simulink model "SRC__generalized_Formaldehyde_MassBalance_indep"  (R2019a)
settings: Solver=VariableStepAuto  StartTime=0.0  StopTime=tend  RelTol=1e-3
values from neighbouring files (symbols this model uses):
  c_MeOH_0 = m_MeOH_sp_0/(m_MeOH_sp_0+m_air_sp_0)    [Mixer_script.m]
  comp_actuator_0 = [z0actuator,comp_w0]    [Compressor_script.m]
  comp_actuator_par = [comp_act_Ga;comp_act_tau;comp_act_zeta]    [Compressor_script.m]
  comp_deltaP = 2.1    [Compressor_script.m]
  comp_p1 = [a0,a1,a2,a3,b0,b1,b2,c0,c1,c2]    [Compressor_script.m]
  comp_p2 = [rho_a, kappa_a, cp_a, R_a, T_amb, d_c]    [Compressor_script.m]
  I_0_compressor = 0.39275    [Compressor_script.m]
  I_0_valve = valve_z0/valve_act_Ga    (= 0.7)    [Valve_script.m]
  Kc_comp = tau_compfotd/(K_compfotd*(tauc_comp+theta_compfotd))    [Compressor_script.m]
  Kc_mtot_MeOH = tau_mtot_MeOH/(K_mtot_MeOH*(tauc_mtot_MeOH+theta_mtot_MeOH))    (= 0.0903815050899)    [Basic_outer_PID_script.m]
  Kc_valve = tau_valvefotd/(K_valvefotd*(tauc_valve+theta_valvefotd))    [Valve_script.m]
  Kc_x_air = tau_x_air/(K_x_air*(tauc_x_air+theta_x_air))    (= -74361.4590706)    [Basic_outer_PID_script.m]
  KI_comp = Kc_comp/tauI_comp    [Compressor_script.m]
  KI_mtot_MeOH = Kc_mtot_MeOH/tauI_mtot_MeOH    [Basic_outer_PID_script.m]
  KI_SRC = Kc_SRC/tauI_SRC    [TuningSRC.m]
  KI_valve = Kc_valve/tauI_valve    [Valve_script.m]
  KI_x_air = Kc_x_air/tauI_x_air    [Basic_outer_PID_script.m]
  m_air_sp_0 = 23920    [Compressor_script.m]
  m_MeOH_sp_0 = 2940    [Valve_script.m]
  m_tot_sp_0 = m_air_sp_0+m_MeOH_sp_0    [main_VPC_formaldehyde.m]    (also in main_basic_formaldehyde.m; main_basicTPM_formaldehyde.m; main_SRC_formaldehyde.m)
  m_tot_sp_step1 = 0*m_tot_sp_0*0.15    [main_VPC_formaldehyde.m]    (also in main_basic_formaldehyde.m; main_basicTPM_formaldehyde.m; main_SRC_formaldehyde.m)
  m_tot_sp_step2 = 1*m_tot_sp_0*0.10    [main_VPC_formaldehyde.m]    (also in main_basic_formaldehyde.m; main_basicTPM_formaldehyde.m; main_SRC_formaldehyde.m)
  m_tot_sp_step3 = 0*(m_tot_sp_step2+m_tot_sp_step1)    [main_VPC_formaldehyde.m]    (also in main_basic_formaldehyde.m = -1*(m_tot_sp_step2+m_tot_sp_step1); main_basicTPM_formaldehyde.m = -1*(m_tot_sp_step2+m_tot_sp_step1); main_SRC_formaldehyde.m = -1*(m_tot_sp_step2+m_tot_sp_step1))
  m_tot_sp_step_t1 = 20    [main_VPC_formaldehyde.m]    (also in main_basic_formaldehyde.m; main_basicTPM_formaldehyde.m; main_SRC_formaldehyde.m)
  m_tot_sp_step_t2 = 30    [main_VPC_formaldehyde.m]    (also in main_basic_formaldehyde.m; main_basicTPM_formaldehyde.m; main_SRC_formaldehyde.m)
  m_tot_sp_step_t3 = 60    [main_VPC_formaldehyde.m]    (also in main_basic_formaldehyde.m = 70; main_basicTPM_formaldehyde.m = 70; main_SRC_formaldehyde.m = 70)
  max_air_PI = mair_max-m_air_sp_0    [Basic_outer_PID_script.m]
  max_MeOH_PI = m_MeOH_max-m_MeOH_sp_0    [Basic_outer_PID_script.m]
  min_air_PI = mair_min-m_air_sp_0    [Basic_outer_PID_script.m]
  min_MeOH_PI = m_MeOH_min-m_MeOH_sp_0    [Basic_outer_PID_script.m]
  N_cmax = 10048    [Compressor_script.m]
  N_cmin = 7500    [Compressor_script.m]
  p_mix = [MW_MeOH;MW_air;rho_MeOH;rho_a;V_mixer]    [Mixer_script.m]
  PI_comp_max = 0.2    [Compressor_script.m]
  PI_comp_min = -I_0_compressor    (= -0.39275)    [Compressor_script.m]
  type_of_bias = 1    [main_SRC_formaldehyde.m]
  valve_actuator_0 = [valve_z0 valve_w0]    [Valve_script.m]
  valve_actuator_par = [valve_act_Ga;valve_act_tau;valve_act_zeta]    [Valve_script.m]
  valve_Cv = m_MeOH_max/sqrt(valve_delta_p)    [Valve_script.m]
  valve_delta_p = 0.5    [Valve_script.m]
  valve_type = 3    [Valve_script.m]
  x_MeOH_sp_step1 = 1*-0.005    (= -0.005)    [main_VPC_formaldehyde.m]    (also in main_basic_formaldehyde.m; main_basicTPM_formaldehyde.m; main_SRC_formaldehyde.m)
  x_MeOH_sp_step2 = 0*-0.005    (= 0)    [main_VPC_formaldehyde.m]    (also in main_basic_formaldehyde.m; main_basicTPM_formaldehyde.m; main_SRC_formaldehyde.m)
  x_MeOH_sp_step3 = 0*+0.01    (= 0)    [main_VPC_formaldehyde.m]    (also in main_basic_formaldehyde.m; main_basicTPM_formaldehyde.m; main_SRC_formaldehyde.m)
  x_MeOH_sp_step_t1 = 10    [main_VPC_formaldehyde.m]    (also in main_basic_formaldehyde.m; main_basicTPM_formaldehyde.m; main_SRC_formaldehyde.m)
  x_MeOH_sp_step_t2 = 40    [main_VPC_formaldehyde.m]    (also in main_basic_formaldehyde.m; main_basicTPM_formaldehyde.m; main_SRC_formaldehyde.m)
  x_MeOH_sp_step_t3 = 60    [main_VPC_formaldehyde.m]    (also in main_basic_formaldehyde.m = 70; main_basicTPM_formaldehyde.m = 70; main_SRC_formaldehyde.m = 70)
  x_MeOHsp_0 = 0.1    [main_VPC_formaldehyde.m]    (also in main_basic_formaldehyde.m; main_basicTPM_formaldehyde.m; main_SRC_formaldehyde.m)
undefined symbols (not defined in the file or in its folder): actuator, Bias_calc, Bias_par, compressor, Kc_air, Kc_MeOH, KI_MeOH, m_MeOH_bias_constant, mixerMeOH_O2_dynamic, mixerMeOH_O2_ss, SRC_par, valve
libraries: simulink x5

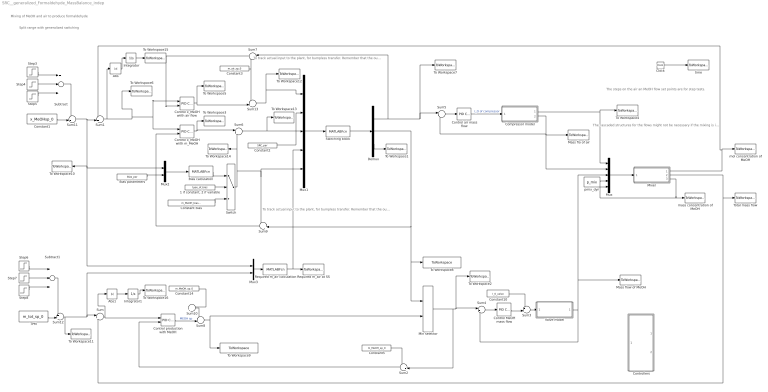
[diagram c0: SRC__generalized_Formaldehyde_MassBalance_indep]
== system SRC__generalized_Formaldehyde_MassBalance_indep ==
  note: Mixing of MeOH and air to produce formaldehyde
  note: The cascaded structures for the flows might not be necessary if the mixing is instantaneous. I just added them to have a general structure. I also added a small residence time in the tank.
  note: The steps on the air an MeOH flow set points are for step tests.
  note: Split range with generalized switching
  note: To track actual input to the plant, for bumpless transfer. Remember that the output of the PI is in deviaton, substract bias.
  note: To track actual input to the plant, for bumpless transfer. Remember that the output of the PI is in deviaton, substract bias.
  "1 if constant, 2 if variable" : Constant  Value=type_of_bias
  Abs : Abs
  Abs1 : Abs
  Bias calculation : MATLABFcn  MATLABFcn=Bias_calc(u)
  Bias parameters : Constant  Value=Bias_par
  Clock : Clock
  Compressor model : Subsystem
  Constant bias : Constant  Value=m_MeOH_bias_constant
  Constant1 : Constant  Value=x_MeOHsp_0
  Constant10 : Constant  Value=I_0_valve
  Constant14 : Constant  Value=m_MeOH_sp_0
  Constant2 : Constant  Value=SRC_par
  Constant3 : Constant  Value=m_air_sp_0
  Constant5 : Constant  Value=m_MeOH_sp_0
  Control MeOH mass flow : simulink/Continuous/PID Controller  Controller=PI  Form=Parallel  TimeDomain=Continuous-time  SampleTime=-1  IntegratorMethod=Forward Euler  FilterMethod=Forward Euler  ControllerParametersSource=internal  P=Kc_valve  I=KI_valve  D=0  UseFilter=on  N=100  TunerSelectOption=Transfer Function Based (PID Tuner App)  InitialConditionSource=internal  InitialConditionForIntegrator=0  InitialConditionForFilter=0  DifferentiatorICPrevScaledInput=0  ExternalReset=none  TrackingMode=off  Kt=1  LimitOutput=on  UpperSaturationLimit=1-I_0_valve  LowerSaturationLimit=-I_0_valve  LinearizeAsGain=on  AntiWindupMode=back-calculation  Kb=1  POutMin=[]  POutMax=[]  IOutMin=[]  IOutMax=[]  DOutMin=[]  DOutMax=[]  NOutMin=[]  NOutMax=[]  SumOutMin=[]  SumOutMax=[]  SaturationOutMin=[]  SaturationOutMax=[]  PParamMin=[]  PParamMax=[]  IParamMin=[]  IParamMax=[]  DParamMin=[]  DParamMax=[]  NParamMin=[]  NParamMax=[]  KbParamMin=[]  KbParamMax=[]  KtParamMin=[]  KtParamMax=[]  KbOutMin=[]  KbOutMax=[]  KtOutMin=[]  KtOutMax=[]  IntegratorOutMin=[]  IntegratorOutMax=[]  FilterOutMin=[]  FilterOutMax=[]  SumI1OutMin=[]  SumI1OutMax=[]  SumI2OutMin=[]  SumI2OutMax=[]  SumI3OutMin=[]  SumI3OutMax=[]  SumI4OutMin=[]  SumI4OutMax=[]  SumDOutMin=[]  SumDOutMax=[]  DifferentiatorOutMin=[]  DifferentiatorOutMax=[]  FilterDiffOutCoefMin=[]  FilterDiffOutCoefMax=[]  ReciprocalOutMin=[]  ReciprocalOutMax=[]  SumDenOutMin=[]  SumDenOutMax=[]  SumNumOutMin=[]  SumNumOutMax=[]  DivideOutMin=[]  DivideOutMax=[]  IntegratorContinuousStateAttributes=''  IntegratorStateMustResolveToSignalObject=off  IntegratorRTWStateStorageClass=Auto  FilterContinuousStateAttributes=''  FilterStateMustResolveToSignalObject=off  FilterRTWStateStorageClass=Auto  ParallelPVariant=InternalParameters  IdealPVariant=Disabled  IVariant=InternalParameters  DVariant=Disabled  IntegratorVariant=Continuous  SatVariant=Enabled  AWVariant=BackCalculation  PCopyVariant=Disabled  TRVariant=Disabled  FdbkBlocksVariant=Forward  IdealPFdbkVariant=Disabled  SatFdbkVariant=Disabled  DerivativeFilterVariant=Disabled  NVariant=Disabled  NCopyVariant=Disabled_SignalSpec  FilterICVariant=Disabled  IntegratorICVariant=InternalICs  ExternalResetVariant=Disabled  TRSumVariant=Passthrough  SumFdbkVariant=Disabled  SumVariant=Sum_PI
  Control air mass flow : simulink/Continuous/PID Controller  Controller=PI  Form=Parallel  TimeDomain=Continuous-time  SampleTime=-1  IntegratorMethod=Forward Euler  FilterMethod=Forward Euler  ControllerParametersSource=internal  P=Kc_comp  I=KI_comp  D=0  UseFilter=on  N=100  TunerSelectOption=Transfer Function Based (PID Tuner App)  InitialConditionSource=internal  InitialConditionForIntegrator=0  InitialConditionForFilter=0  DifferentiatorICPrevScaledInput=0  ExternalReset=none  TrackingMode=off  Kt=1  LimitOutput=on  UpperSaturationLimit=PI_comp_max  LowerSaturationLimit=PI_comp_min  LinearizeAsGain=on  AntiWindupMode=back-calculation  Kb=1  POutMin=[]  POutMax=[]  IOutMin=[]  IOutMax=[]  DOutMin=[]  DOutMax=[]  NOutMin=[]  NOutMax=[]  SumOutMin=[]  SumOutMax=[]  SaturationOutMin=[]  SaturationOutMax=[]  PParamMin=[]  PParamMax=[]  IParamMin=[]  IParamMax=[]  DParamMin=[]  DParamMax=[]  NParamMin=[]  NParamMax=[]  KbParamMin=[]  KbParamMax=[]  KtParamMin=[]  KtParamMax=[]  KbOutMin=[]  KbOutMax=[]  KtOutMin=[]  KtOutMax=[]  IntegratorOutMin=[]  IntegratorOutMax=[]  FilterOutMin=[]  FilterOutMax=[]  SumI1OutMin=[]  SumI1OutMax=[]  SumI2OutMin=[]  SumI2OutMax=[]  SumI3OutMin=[]  SumI3OutMax=[]  SumI4OutMin=[]  SumI4OutMax=[]  SumDOutMin=[]  SumDOutMax=[]  DifferentiatorOutMin=[]  DifferentiatorOutMax=[]  FilterDiffOutCoefMin=[]  FilterDiffOutCoefMax=[]  ReciprocalOutMin=[]  ReciprocalOutMax=[]  SumDenOutMin=[]  SumDenOutMax=[]  SumNumOutMin=[]  SumNumOutMax=[]  DivideOutMin=[]  DivideOutMax=[]  IntegratorContinuousStateAttributes=''  IntegratorStateMustResolveToSignalObject=off  IntegratorRTWStateStorageClass=Auto  FilterContinuousStateAttributes=''  FilterStateMustResolveToSignalObject=off  FilterRTWStateStorageClass=Auto  ParallelPVariant=InternalParameters  IdealPVariant=Disabled  IVariant=InternalParameters  DVariant=Disabled  IntegratorVariant=Continuous  SatVariant=Enabled  AWVariant=BackCalculation  PCopyVariant=Disabled  TRVariant=Disabled  FdbkBlocksVariant=Forward  IdealPFdbkVariant=Disabled  SatFdbkVariant=Disabled  DerivativeFilterVariant=Disabled  NVariant=Disabled  NCopyVariant=Disabled_SignalSpec  FilterICVariant=Disabled  IntegratorICVariant=InternalICs  ExternalResetVariant=Disabled  TRSumVariant=Passthrough  SumFdbkVariant=Disabled  SumVariant=Sum_PI
  Control production with MeOH : simulink/Continuous/PID Controller  Controller=PI  Form=Parallel  TimeDomain=Continuous-time  SampleTime=-1  IntegratorMethod=Forward Euler  FilterMethod=Forward Euler  ControllerParametersSource=internal  P=Kc_mtot_MeOH  I=KI_mtot_MeOH  D=0  UseFilter=on  N=100  TunerSelectOption=Transfer Function Based (PID Tuner App)  InitialConditionSource=internal  InitialConditionForIntegrator=0  InitialConditionForFilter=0  DifferentiatorICPrevScaledInput=0  ExternalReset=none  TrackingMode=on  Kt=1  LimitOutput=on  UpperSaturationLimit=max_MeOH_PI  LowerSaturationLimit=min_MeOH_PI  LinearizeAsGain=on  AntiWindupMode=back-calculation  Kb=1  POutMin=[]  POutMax=[]  IOutMin=[]  IOutMax=[]  DOutMin=[]  DOutMax=[]  NOutMin=[]  NOutMax=[]  SumOutMin=[]  SumOutMax=[]  SaturationOutMin=[]  SaturationOutMax=[]  PParamMin=[]  PParamMax=[]  IParamMin=[]  IParamMax=[]  DParamMin=[]  DParamMax=[]  NParamMin=[]  NParamMax=[]  KbParamMin=[]  KbParamMax=[]  KtParamMin=[]  KtParamMax=[]  KbOutMin=[]  KbOutMax=[]  KtOutMin=[]  KtOutMax=[]  IntegratorOutMin=[]  IntegratorOutMax=[]  FilterOutMin=[]  FilterOutMax=[]  SumI1OutMin=[]  SumI1OutMax=[]  SumI2OutMin=[]  SumI2OutMax=[]  SumI3OutMin=[]  SumI3OutMax=[]  SumI4OutMin=[]  SumI4OutMax=[]  SumDOutMin=[]  SumDOutMax=[]  DifferentiatorOutMin=[]  DifferentiatorOutMax=[]  FilterDiffOutCoefMin=[]  FilterDiffOutCoefMax=[]  ReciprocalOutMin=[]  ReciprocalOutMax=[]  SumDenOutMin=[]  SumDenOutMax=[]  SumNumOutMin=[]  SumNumOutMax=[]  DivideOutMin=[]  DivideOutMax=[]  IntegratorContinuousStateAttributes=''  IntegratorStateMustResolveToSignalObject=off  IntegratorRTWStateStorageClass=Auto  FilterContinuousStateAttributes=''  FilterStateMustResolveToSignalObject=off  FilterRTWStateStorageClass=Auto  ParallelPVariant=InternalParameters  IdealPVariant=Disabled  IVariant=InternalParameters  DVariant=Disabled  IntegratorVariant=Continuous  SatVariant=Enabled  AWVariant=BackCalculation  PCopyVariant=Disabled  TRVariant=Enabled  FdbkBlocksVariant=Forward  IdealPFdbkVariant=Disabled  SatFdbkVariant=Disabled  DerivativeFilterVariant=Disabled  NVariant=Disabled  NCopyVariant=Disabled_SignalSpec  FilterICVariant=Disabled  IntegratorICVariant=InternalICs  ExternalResetVariant=Disabled  TRSumVariant=TrackingMode  SumFdbkVariant=Disabled  SumVariant=Sum_PI
  Control x_MeOH wiith air flow : simulink/Continuous/PID Controller  Controller=PI  Form=Parallel  TimeDomain=Continuous-time  SampleTime=-1  IntegratorMethod=Forward Euler  FilterMethod=Forward Euler  ControllerParametersSource=internal  P=Kc_x_air  I=KI_x_air  D=0  UseFilter=on  N=100  TunerSelectOption=Transfer Function Based (PID Tuner App)  InitialConditionSource=internal  InitialConditionForIntegrator=0  InitialConditionForFilter=0  DifferentiatorICPrevScaledInput=0  ExternalReset=none  TrackingMode=on  Kt=1  LimitOutput=on  UpperSaturationLimit=max_air_PI  LowerSaturationLimit=min_air_PI  LinearizeAsGain=on  AntiWindupMode=back-calculation  Kb=1  POutMin=[]  POutMax=[]  IOutMin=[]  IOutMax=[]  DOutMin=[]  DOutMax=[]  NOutMin=[]  NOutMax=[]  SumOutMin=[]  SumOutMax=[]  SaturationOutMin=[]  SaturationOutMax=[]  PParamMin=[]  PParamMax=[]  IParamMin=[]  IParamMax=[]  DParamMin=[]  DParamMax=[]  NParamMin=[]  NParamMax=[]  KbParamMin=[]  KbParamMax=[]  KtParamMin=[]  KtParamMax=[]  KbOutMin=[]  KbOutMax=[]  KtOutMin=[]  KtOutMax=[]  IntegratorOutMin=[]  IntegratorOutMax=[]  FilterOutMin=[]  FilterOutMax=[]  SumI1OutMin=[]  SumI1OutMax=[]  SumI2OutMin=[]  SumI2OutMax=[]  SumI3OutMin=[]  SumI3OutMax=[]  SumI4OutMin=[]  SumI4OutMax=[]  SumDOutMin=[]  SumDOutMax=[]  DifferentiatorOutMin=[]  DifferentiatorOutMax=[]  FilterDiffOutCoefMin=[]  FilterDiffOutCoefMax=[]  ReciprocalOutMin=[]  ReciprocalOutMax=[]  SumDenOutMin=[]  SumDenOutMax=[]  SumNumOutMin=[]  SumNumOutMax=[]  DivideOutMin=[]  DivideOutMax=[]  IntegratorContinuousStateAttributes=''  IntegratorStateMustResolveToSignalObject=off  IntegratorRTWStateStorageClass=Auto  FilterContinuousStateAttributes=''  FilterStateMustResolveToSignalObject=off  FilterRTWStateStorageClass=Auto  ParallelPVariant=InternalParameters  IdealPVariant=Disabled  IVariant=InternalParameters  DVariant=Disabled  IntegratorVariant=Continuous  SatVariant=Enabled  AWVariant=BackCalculation  PCopyVariant=Disabled  TRVariant=Enabled  FdbkBlocksVariant=Forward  IdealPFdbkVariant=Disabled  SatFdbkVariant=Disabled  DerivativeFilterVariant=Disabled  NVariant=Disabled  NCopyVariant=Disabled_SignalSpec  FilterICVariant=Disabled  IntegratorICVariant=InternalICs  ExternalResetVariant=Disabled  TRSumVariant=TrackingMode  SumFdbkVariant=Disabled  SumVariant=Sum_PI
  Control x_MeOH wiith m_MeOH : simulink/Continuous/PID Controller  Controller=PI  Form=Parallel  TimeDomain=Continuous-time  SampleTime=-1  IntegratorMethod=Forward Euler  FilterMethod=Forward Euler  ControllerParametersSource=internal  P=Kc_MeOH  I=KI_MeOH  D=0  UseFilter=on  N=100  TunerSelectOption=Transfer Function Based (PID Tuner App)  InitialConditionSource=internal  InitialConditionForIntegrator=0  InitialConditionForFilter=0  DifferentiatorICPrevScaledInput=0  ExternalReset=none  TrackingMode=on  Kt=1  LimitOutput=on  UpperSaturationLimit=inf  LowerSaturationLimit=-inf  LinearizeAsGain=on  AntiWindupMode=back-calculation  Kb=1  POutMin=[]  POutMax=[]  IOutMin=[]  IOutMax=[]  DOutMin=[]  DOutMax=[]  NOutMin=[]  NOutMax=[]  SumOutMin=[]  SumOutMax=[]  SaturationOutMin=[]  SaturationOutMax=[]  PParamMin=[]  PParamMax=[]  IParamMin=[]  IParamMax=[]  DParamMin=[]  DParamMax=[]  NParamMin=[]  NParamMax=[]  KbParamMin=[]  KbParamMax=[]  KtParamMin=[]  KtParamMax=[]  KbOutMin=[]  KbOutMax=[]  KtOutMin=[]  KtOutMax=[]  IntegratorOutMin=[]  IntegratorOutMax=[]  FilterOutMin=[]  FilterOutMax=[]  SumI1OutMin=[]  SumI1OutMax=[]  SumI2OutMin=[]  SumI2OutMax=[]  SumI3OutMin=[]  SumI3OutMax=[]  SumI4OutMin=[]  SumI4OutMax=[]  SumDOutMin=[]  SumDOutMax=[]  DifferentiatorOutMin=[]  DifferentiatorOutMax=[]  FilterDiffOutCoefMin=[]  FilterDiffOutCoefMax=[]  ReciprocalOutMin=[]  ReciprocalOutMax=[]  SumDenOutMin=[]  SumDenOutMax=[]  SumNumOutMin=[]  SumNumOutMax=[]  DivideOutMin=[]  DivideOutMax=[]  IntegratorContinuousStateAttributes=''  IntegratorStateMustResolveToSignalObject=off  IntegratorRTWStateStorageClass=Auto  FilterContinuousStateAttributes=''  FilterStateMustResolveToSignalObject=off  FilterRTWStateStorageClass=Auto  ParallelPVariant=InternalParameters  IdealPVariant=Disabled  IVariant=InternalParameters  DVariant=Disabled  IntegratorVariant=Continuous  SatVariant=Enabled  AWVariant=BackCalculation  PCopyVariant=Disabled  TRVariant=Enabled  FdbkBlocksVariant=Forward  IdealPFdbkVariant=Disabled  SatFdbkVariant=Disabled  DerivativeFilterVariant=Disabled  NVariant=Disabled  NCopyVariant=Disabled_SignalSpec  FilterICVariant=Disabled  IntegratorICVariant=InternalICs  ExternalResetVariant=Disabled  TRSumVariant=TrackingMode  SumFdbkVariant=Disabled  SumVariant=Sum_PI
  Controllers : Subsystem
  Demux : Demux  Outputs=3
  Integrator : Integrator
  Integrator1 : Integrator
  Mass flo of air : ToWorkspace  VariableName=m_air  SampleTime=-1
  Mass flow of MeOH : ToWorkspace  VariableName=m_MeOH  SampleTime=-1
  Min selector : MinMax  Inputs=2
  Mixer : Subsystem
  Mux : Mux  Inputs=5
  Mux1 : Mux  Inputs=5
  Mux2 : Mux  Inputs=2
  Mux3 : Mux  Inputs=2
  Required m_air at SS : ToWorkspace  VariableName=m_air_req  SampleTime=-1
  Required m_air calculation : MATLABFcn  MATLABFcn=Required_mair  OutputDimensions=1
  Step3 : Step  Time=x_MeOH_sp_step_t1  After=x_MeOH_sp_step1  SampleTime=0
  Step4 : Step  Time=x_MeOH_sp_step_t2  After=x_MeOH_sp_step2  SampleTime=0
  Step5 : Step  Time=x_MeOH_sp_step_t3  After=x_MeOH_sp_step3  SampleTime=0
  Step6 : Step  Time=m_tot_sp_step_t1  After=m_tot_sp_step1  SampleTime=0
  Step7 : Step  Time=m_tot_sp_step_t2  After=m_tot_sp_step2  SampleTime=0
  Step8 : Step  Time=m_tot_sp_step_t3  After=m_tot_sp_step3  SampleTime=0
  Subtract : Sum  Inputs=+++
  Subtract1 : Sum  Inputs=+++
  Sum{,4..5,7} (4 alike) : Sum  Inputs=|+-
  Sum1 : Sum  Inputs=-+|
  Sum{3,8,10..13} (6 alike) : Sum  Inputs=++|
  Sum2 : Sum  Inputs=-+|
  Sum6 : Sum  Inputs=|++
  Sum9 : Sum  Inputs=-+|
  Switch : Switch  Criteria=u2 > Threshold  Threshold=1
  Switching block : MATLABFcn  MATLABFcn=SR_switch2_MassBalance  OutputDimensions=3
  TPM : Constant  Value=m_tot_sp_0
  To Workspace1 : ToWorkspace  VariableName=activeMV  SampleTime=-1
  To Workspace10 : ToWorkspace  VariableName=x_MeOHsp  SampleTime=-1
  To Workspace11 : ToWorkspace  VariableName=m_tot_sp  SampleTime=-1
  To Workspace12 : ToWorkspace  VariableName=u_air  SampleTime=-1
  To Workspace13 : ToWorkspace  VariableName=u_MeOH  SampleTime=-1
  To Workspace14 : ToWorkspace  VariableName=bias_MeOH  SampleTime=-1
  To Workspace15 : ToWorkspace  VariableName=IAE_xMeOH  SampleTime=-1
  To Workspace16 : ToWorkspace  VariableName=IAE_mtot  SampleTime=-1
  To Workspace2 : ToWorkspace  VariableName=m_MEOH_sp  SampleTime=-1
  To Workspace3 : ToWorkspace  VariableName=v_MeOH  SampleTime=-1
  To Workspace4 : ToWorkspace  VariableName=Q_air  SampleTime=-1
  To Workspace5 : ToWorkspace  VariableName=v_air  SampleTime=-1
  To Workspace6 : ToWorkspace  VariableName=x_MeOH_error  SampleTime=-1
  To Workspace7 : ToWorkspace  VariableName=m_air_sp  SampleTime=-1
  To Workspace8 : ToWorkspace  VariableName=m_MEOH_sp_SR  SampleTime=-1
  To Workspace9 : ToWorkspace  VariableName=m_MeOH_sp_m_tot  SampleTime=-1
  Total mass flow : ToWorkspace  VariableName=m_tot  SampleTime=-1
  Valve model : Subsystem
  mass concentration of MeOH : ToWorkspace  VariableName=c_MeOH  SampleTime=-1
  mol concentration of MeOH : ToWorkspace  VariableName=x_MeOH  SampleTime=-1
  pmix_dyn : Constant  Value=p_mix
  time : ToWorkspace  VariableName=t  SampleTime=-1
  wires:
  Valve model/1(m_MeOH) -> Mass flow of MeOH/1, Mux/3, Sum4/2
  Clock/1 -> time/1
  Compressor model/2(m_air) -> Sum5/2, Mux/2, Mass flo of air/1
  Compressor model/1(Q_air) -> Mux/1, To Workspace4/1
  Control MeOH mass flow/1 -> Sum3/2
  Constant10/1 -> Sum3/1
  Sum4/1 -> Control MeOH mass flow/1
  Mixer/2(m_tot) -> Total mass flow/1, Sum/2
  Mixer/1(x_MeOH) -> Sum1/1, mol concentration of MeOH/1
  pmix_dyn/1 -> Mux/4
  Sum10/1 -> Sum8/1
  Constant1/1 -> Sum11/2
  Sum11/1 -> Mux3/1, Mux2/1, To Workspace10/1, Sum1/2
  Step3/1 -> Subtract/1
  Step4/1 -> Subtract/2
  Step5/1 -> Subtract/3
  TPM/1 -> Sum12/2
  Sum12/1 -> To Workspace11/1, Mux3/2, Sum/1
  Step6/1 -> Subtract1/1
  Step7/1 -> Subtract1/2
  Step8/1 -> Subtract1/3
  Subtract1/1 -> Sum12/1
  Sum1/1 -> Abs/1, Control x_MeOH wiith m_MeOH/1, Control x_MeOH wiith air flow/1, To Workspace6/1
  Control air mass flow/1 -> Compressor model/1(I_blower)  "I_O of compressor"
  Sum5/1 -> Control air mass flow/1
  Mux/1 -> Mixer/1(Mix_par)
  Mixer/3(c_MeOH) -> Mux/5, mass concentration of MeOH/1
  Sum3/1 -> Valve model/1(I_valve)
  Mux1/1 -> Switching block/1
  Control x_MeOH wiith air flow/1 -> Sum13/2, To Workspace5/1
  Control x_MeOH wiith m_MeOH/1 -> To Workspace3/1, Sum6/1
  Switching block/1 -> Demux/1
  Demux/3 -> To Workspace1/1
  Demux/2 -> Sum9/2, Min selector/1, To Workspace8/1
  Sum/1 -> Abs1/1, Control production with MeOH/1
  Sum8/1 -> To Workspace9/1, Min selector/2
  Min selector/1 -> Sum2/2, To Workspace2/1, Sum4/1
  Sum13/1 -> To Workspace12/1, Mux1/1
  Constant3/1 -> Sum13/1, Sum7/2
  Sum6/1 -> To Workspace13/1, Mux1/2
  Constant2/1 -> Mux1/3
  Constant14/1 -> Sum10/1
  Constant bias/1 -> Switch/3
  Switch/1 -> Mux1/5, Sum9/1, To Workspace14/1, Sum6/2
  "1 if constant, 2 if variable"/1 -> Switch/2
  Bias calculation/1 -> Switch/1
  Mux2/1 -> Bias calculation/1
  Bias parameters/1 -> Mux2/2
  Demux/1 -> Sum7/1, To Workspace7/1, Sum5/1
  Control production with MeOH/1 -> Sum8/2  "MEOH sp"
  Subtract/1 -> Sum11/1
  Required m_air calculation/1 -> Required m_air at SS/1, Mux1/4
  Mux3/1 -> Required m_air calculation/1
  Constant5/1 -> Sum2/1
  Sum2/1 -> Control production with MeOH/2
  Sum7/1 -> Control x_MeOH wiith air flow/2
  Sum9/1 -> Control x_MeOH wiith m_MeOH/2
  Abs/1 -> Integrator/1
  Integrator/1 -> To Workspace15/1
  Abs1/1 -> Integrator1/1
  Integrator1/1 -> To Workspace16/1

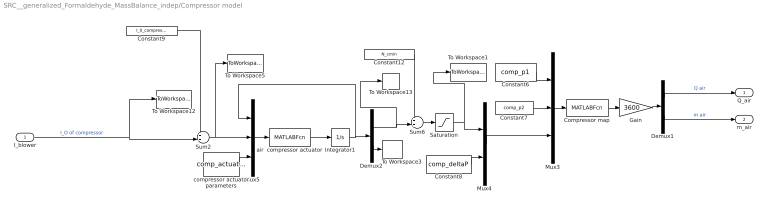
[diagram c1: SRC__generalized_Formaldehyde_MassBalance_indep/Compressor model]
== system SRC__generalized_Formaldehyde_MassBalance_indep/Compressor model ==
  I_blower : Inport
  Compressor map : MATLABFcn  MATLABFcn=compressor(u(1:10),u(11:16),u(17:18))  OutputDimensions=2
  Constant12 : Constant  Value=N_cmin
  Constant6 : Constant  Value=comp_p1
  Constant7 : Constant  Value=comp_p2
  Constant8 : Constant  Value=comp_deltaP
  Constant9 : Constant  Value=I_0_compressor
  Demux1 : Demux  Outputs=2
  Demux2 : Demux  Outputs=2
  Gain : Gain  Gain=3600
  Integrator1 : Integrator  InitialCondition=comp_actuator_0
  Mux3 : Mux  Inputs=3
  Mux4 : Mux  Inputs=2
  Mux5 : Mux  Inputs=3
  Saturation : Saturate  UpperLimit=N_cmax  LowerLimit=N_cmin
  Sum2 : Sum  Inputs=++|
  Sum6 : Sum  Inputs=++|
  To Workspace1 : ToWorkspace  VariableName=comp_rpm  SampleTime=-1
  To Workspace12 : ToWorkspace  VariableName=I_air0  SampleTime=-1
  To Workspace13 : ToWorkspace  VariableName=Nc_act1  SampleTime=-1
  To Workspace3 : ToWorkspace  VariableName=wcomp  SampleTime=-1
  To Workspace5 : ToWorkspace  VariableName=I_air  SampleTime=-1
  air  compressor actuator : MATLABFcn  MATLABFcn=actuator(u(1:2),u(3),u(4:6))  OutputDimensions=2
  compressor actuator parameters : Constant  Value=comp_actuator_par
  Q_air : Outport
  m_air : Outport  Port=2
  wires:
  I_blower/1 -> To Workspace12/1, Sum2/2  "I_O of compressor"
  Constant9/1 -> Sum2/1
  Sum6/1 -> Saturation/1
  Constant12/1 -> Sum6/1
  Constant6/1 -> Mux3/1
  Mux5/1 -> air  compressor actuator/1
  Sum2/1 -> To Workspace5/1, Mux5/2
  Integrator1/1 -> Demux2/1, Mux5/1
  Demux2/1 -> To Workspace13/1, Sum6/2
  air  compressor actuator/1 -> Integrator1/1
  Constant8/1 -> Mux4/2
  Demux2/2 -> To Workspace3/1
  Demux1/1 -> Q_air/1  "Q air"
  Mux3/1 -> Compressor map/1
  Constant7/1 -> Mux3/2
  Mux4/1 -> Mux3/3
  Saturation/1 -> To Workspace1/1, Mux4/1
  Compressor map/1 -> Gain/1
  Gain/1 -> Demux1/1
  Demux1/2 -> m_air/1  "m air"
  compressor actuator parameters/1 -> Mux5/3

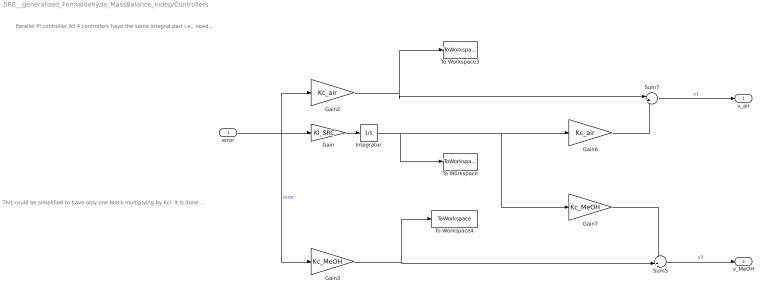
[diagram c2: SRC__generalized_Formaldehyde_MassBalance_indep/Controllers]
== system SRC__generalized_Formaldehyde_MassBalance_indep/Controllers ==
  note: Parallel PI controller All 4 controllers have the same integral part i.e., need Ki=Kc\tauI equal for all processes consider Tsp=Tamb, then all MV are closed, so the nominal point for all MVs is 0.
  note: This could be simplified to have only one block multiplying by Kci. It is done separately to have the value of Kc*error and understand better what is happening
  error : Inport
  Gain : Gain  Gain=KI_SRC
  Gain2 : Gain  Gain=Kc_air
  Gain3 : Gain  Gain=Kc_MeOH
  Gain6 : Gain  Gain=Kc_air
  Gain7 : Gain  Gain=Kc_MeOH
  Integrator : Integrator
  Sum5 : Sum  Inputs=++|
  Sum7 : Sum  Inputs=|++
  To Workspace : ToWorkspace  VariableName=integral  SampleTime=-1
  To Workspace3 : ToWorkspace  VariableName=Kce_air  SampleTime=-1
  To Workspace4 : ToWorkspace  VariableName=Kce_MeOH  SampleTime=-1
  v_air : Outport
  v_MeOH : Outport  Port=2
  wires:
  Integrator/1 -> To Workspace/1, Gain7/1, Gain6/1
  Gain/1 -> Integrator/1
  Gain2/1 -> Sum7/1, To Workspace3/1
  error/1 -> Gain3/1, Gain/1, Gain2/1  "error"
  Sum7/1 -> v_air/1  "v1"
  Sum5/1 -> v_MeOH/1  "v2"
  Gain3/1 -> To Workspace4/1, Sum5/2
  Gain7/1 -> Sum5/1
  Gain6/1 -> Sum7/2

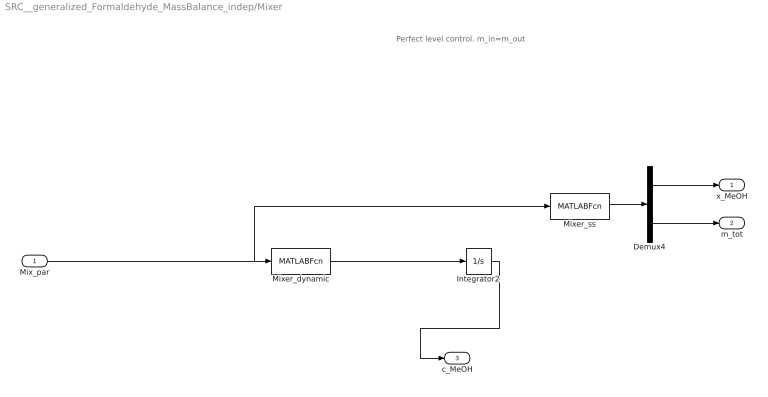
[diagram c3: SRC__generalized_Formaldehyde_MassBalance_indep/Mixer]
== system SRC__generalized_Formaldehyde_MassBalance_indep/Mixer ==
  note: Perfect level control. m_in=m_out
  Mix_par : Inport
  Demux4 : Demux  Outputs=2
  Integrator2 : Integrator  InitialCondition=c_MeOH_0
  Mixer_dynamic : MATLABFcn  MATLABFcn=mixerMeOH_O2_dynamic(u(1:3),u(4:8),u(9))  OutputDimensions=1
  Mixer_ss : MATLABFcn  MATLABFcn=mixerMeOH_O2_ss(u(1:3),u(4:8),u(9))  OutputDimensions=2
  x_MeOH : Outport
  m_tot : Outport  Port=2
  c_MeOH : Outport  Port=3
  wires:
  Integrator2/1 -> c_MeOH/1
  Mix_par/1 -> Mixer_ss/1, Mixer_dynamic/1
  Mixer_dynamic/1 -> Integrator2/1
  Mixer_ss/1 -> Demux4/1
  Demux4/1 -> x_MeOH/1
  Demux4/2 -> m_tot/1

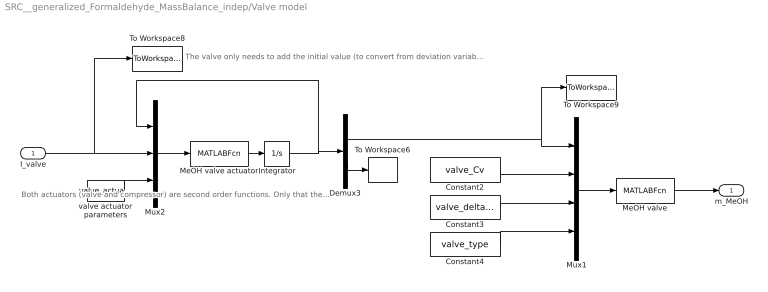
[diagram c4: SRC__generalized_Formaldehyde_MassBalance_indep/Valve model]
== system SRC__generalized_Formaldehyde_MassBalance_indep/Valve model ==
  note: The valve only needs to add the initial value (to convert from deviation variables to actual variables "once" before the actuator. The compressor also needs it before the actuator because the range does not start in 0. (Maybe there is a better way to do this).
  note: Both actuators (valve and compressor) are second order functions. Only that the time constants and the damping factors are different.
  I_valve : Inport
  Constant2 : Constant  Value=valve_Cv
  Constant3 : Constant  Value=valve_delta_p
  Constant4 : Constant  Value=valve_type
  Demux3 : Demux  Outputs=2
  Integrator : Integrator  InitialCondition=valve_actuator_0
  MeOH valve : MATLABFcn  MATLABFcn=valve(u)  OutputDimensions=1
  MeOH valve actuator : MATLABFcn  MATLABFcn=actuator(u(1:2),u(3),u(4:6))  OutputDimensions=2
  Mux1 : Mux
  Mux2 : Mux  Inputs=3
  To Workspace6 : ToWorkspace  VariableName=wvalve  SampleTime=-1
  To Workspace8 : ToWorkspace  VariableName=I_MeOH  SampleTime=-1
  To Workspace9 : ToWorkspace  VariableName=z_MeOH  SampleTime=-1
  valve actuator parameters : Constant  Value=valve_actuator_par
  m_MeOH : Outport
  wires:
  Demux3/2 -> To Workspace6/1
  Demux3/1 -> To Workspace9/1, Mux1/1
  MeOH valve actuator/1 -> Integrator/1
  Integrator/1 -> Demux3/1, Mux2/1
  Constant4/1 -> Mux1/4
  Constant3/1 -> Mux1/3
  I_valve/1 -> To Workspace8/1, Mux2/2
  Constant2/1 -> Mux1/2
  Mux2/1 -> MeOH valve actuator/1
  Mux1/1 -> MeOH valve/1
  valve actuator parameters/1 -> Mux2/3
  MeOH valve/1 -> m_MeOH/1
